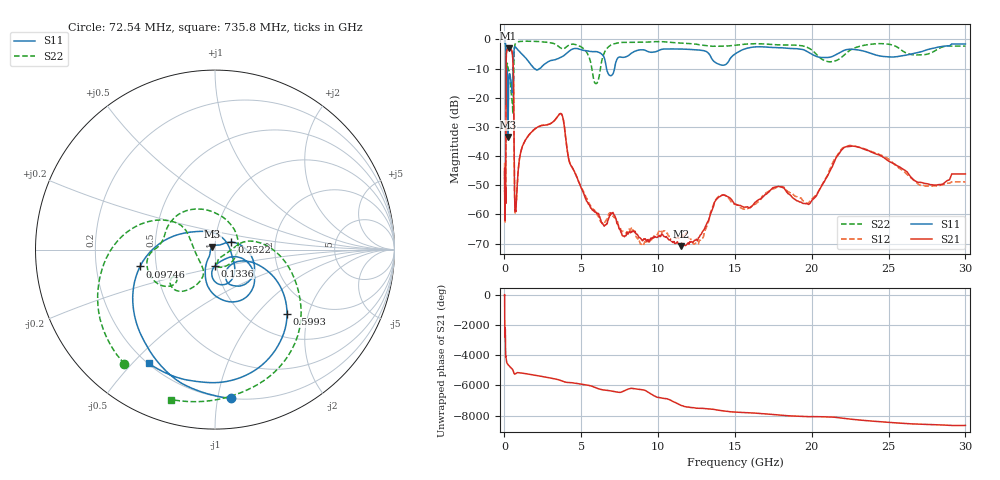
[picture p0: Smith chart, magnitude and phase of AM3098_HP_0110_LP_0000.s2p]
! Date/Time: Thu, Feb 28, 2019 8:37 AM
! Network Analyzer: Agilent Technologies E8364B Rev: A.07.50.67
! Sweep from 0.010 to 30.000 GHz, 1601 Points, Sweep Type: LOG
! Power Supply: 5.023 V, 0.002 A
# Hz S DB R 50
!freq MagS11 AngS11 MagS21 AngS21 MagS12 AngS12 MagS22 AngS22
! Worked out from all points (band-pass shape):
!   1601 points, 10 MHz to 30 GHz, reference 50 ohm
!   highest |S21| = -2.98 dB at 266.5 MHz (marker M1); lowest = -70.9 dB at 11.48 GHz (marker M2)
!   |S21| within 3 dB of the highest: 117.3 MHz to 534.3 MHz (417 MHz wide, 128 % of centre)
!   lowest |S11| = -33.4 dB at 231.6 MHz (marker M3), VSWR 1.04, Z = 48.5 + j1.5 ohm
!   |S11| at or under -10 dB: 175.5 MHz to 562.4 MHz (386.9 MHz wide, 105 % of centre); 1.96 GHz to 2.28 GHz (319.8 MHz wide, 15.1 % of centre); 6.644 GHz to 7.165 GHz (520.8 MHz wide, 7.54 % of centre)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
!   |S22| runs from -25.5 to -0.5 dB; largest |S21 - S12| = 0.011
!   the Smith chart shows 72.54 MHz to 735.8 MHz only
!   S11 on the Smith chart (normalised r, x): 72.54 MHz: 0.20, -1.09; 97.46 MHz: 0.40, -0.09; 133.6 MHz: 0.99, -0.18; 252.2 MHz: 1.20, +0.10; 599.3 MHz: 1.45, -1.48; 735.8 MHz: 0.20, -0.56
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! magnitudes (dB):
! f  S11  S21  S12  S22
! 10 MHz  -0.3  -47.7  -42.4  -0.5
! 38.04 MHz  -0.5  -57.6  -58.2  -0.7
! 72.54 MHz  -1.6  -52.5  -51.3  -1.8
! 84.71 MHz  -2.7  -50.0  -50.2  -2.9
! 97.46 MHz  -7.4  -23.6  -23.5  -8.7
! 133.6 MHz  -21.0  -4.4  -4.4  -11.0
! 144.7 MHz  -18.8  -3.9  -3.8  -11.2
! 186.8 MHz  -11.0  -3.5  -3.5  -8.2
! 231.6 MHz  -33.4  -3.1  -3.1  -10.1
! 252.2 MHz  -20.0  -3.0  -3.0  -10.5
! 266.5 MHz  -16.0  -3.0  -2.9  -10.7
! 550.5 MHz  -12.0  -7.2  -7.2  -25.3
! 599.3 MHz  -5.4  -18.4  -18.4  -10.0
! 669.1 MHz  -2.6  -55.9  -56.7  -2.2
! 735.8 MHz  -2.7  -58.8  -57.7  -1.2
! 2.084 GHz  -10.4  -30.3  -30.3  -0.7
! 3.686 GHz  -6.1  -25.5  -25.4  -3.0
! 5.959 GHz  -4.2  -59.2  -59.3  -15.2
! 7.926 GHz  -5.9  -67.2  -66.3  -1.0
! 11.48 GHz  -3.3  -70.9  -67.4  -1.3
! 22.67 GHz  -3.4  -36.6  -36.5  -3.2
! 30 GHz  -1.6  -46.1  -48.8  -2.3
